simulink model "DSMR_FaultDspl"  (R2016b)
settings: Solver=FixedStepDiscrete  StartTime=0.0  StopTime=10.0  FixedStep=0.02  RelTol=1e-3  EnableMultiTasking=on
undefined symbols (not defined in the file): bin2dec
libraries: simulink x312
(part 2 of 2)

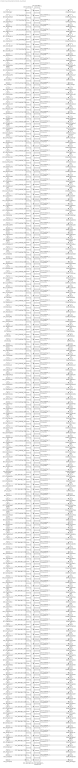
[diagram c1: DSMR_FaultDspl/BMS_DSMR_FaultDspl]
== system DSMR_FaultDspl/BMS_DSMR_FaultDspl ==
  DFC_CurrRngErr : Inport
  DFC_BattVoltRngErr : Inport  Port=2
  DFC_BattHVMsgTmt : Inport  Port=3
  DFC_BusHVMsgTmt : Inport  Port=4
  DFC_638LinCommErr : Inport  Port=5
  DFC_CellTempTmt : Inport  Port=6
  DFC_CellVoltTmt : Inport  Port=7
  DFC_InCanBusOff : Inport  Port=8
  DFC_VeCanBusOff : Inport  Port=9
  DFC_Msg2A3Tmt : Inport  Port=10
  DFC_RcMsg2A3Mis : Inport  Port=11
  DFC_ChkSumMsg2A3Err : Inport  Port=12
  DFC_RcMsg2A5Mis : Inport  Port=13
  DFC_RcMsg2A7Mis : Inport  Port=14
  DFC_CrashNpl : Inport  Port=15
  DFC_FuseNpl : Inport  Port=16
  DFC_Kl30cVoltLoErr : Inport  Port=17
  DFC_PosStuckMax : Inport  Port=18
  DFC_MPosStuckMin : Inport  Port=19
  DFC_MNegStuckMax : Inport  Port=20
  DFC_MNegStuckMin : Inport  Port=21
  DFC_PrStuckMin : Inport  Port=22
  DFC_DChrgPosStuckMax : Inport  Port=23
  DFC_DChrgPosStuckMin : Inport  Port=24
  DFC_DChrgNegStuckMax : Inport  Port=25
  DFC_DChrgNegStuckMin : Inport  Port=26
  DFC_HvPwrUpFail : Inport  Port=27
  DFC_DChrgPwrUpFail : Inport  Port=28
  DFC_BattTAlrmMax : Inport  Port=29
  DFC_BattTFaultMax : Inport  Port=30
  DFC_BattTAlrmMin : Inport  Port=31
  DFC_BattTFaultMin : Inport  Port=32
  DFC_BattTempVldMin : Inport  Port=33
  DFC_BattTCnstMax : Inport  Port=34
  DFC_BattTGradtMax : Inport  Port=35
  DFC_CellVoltAlrmMax : Inport  Port=36
  DFC_CellVoltFaultMax : Inport  Port=37
  DFC_CellVoltFusfMax : Inport  Port=38
  DFC_CellVoltAlrmMin : Inport  Port=39
  DFC_CellVoltFusfMin : Inport  Port=40
  DFC_CellVoltFaultMin : Inport  Port=41
  DFC_CellVoltVldMin : Inport  Port=42
  DFC_CellVoltNpl : Inport  Port=43
  DFC_Msg2E6Tmt : Inport  Port=44
  DFC_RcMsg2E6Mis : Inport  Port=45
  DFC_ChkSumMsg2E6Err : Inport  Port=46
  DFC_RcMsg2E1Mis : Inport  Port=47
  DFC_ChkSumMsg2E1Err : Inport  Port=48
  DFC_DcCanBusOff : Inport  Port=49
  DFC_DChrgTCnntMax : Inport  Port=50
  DFC_ChrgOCNpl : Inport  Port=51
  DFC_DisChOCNpl : Inport  Port=52
  DFC_BattVoltHiMax : Inport  Port=53
  DFC_BattVoltLoMin : Inport  Port=54
  DFC_ThmRnwy : Inport  Port=55
  DFC_AChrgPortOvrTemp : Inport  Port=56
  DFC_CurrOffsPlaus : Inport  Port=57
  DFC_CurrStukPlaus : Inport  Port=58
  DFC_CurrChrgPlaus : Inport  Port=59
  DFC_BattUNpl : Inport  Port=60
  DFC_BattVoltVld : Inport  Port=61
  DFC_PackUNpl : Inport  Port=62
  DFC_PackVoltVld : Inport  Port=63
  DFC_DChrgUNpl : Inport  Port=64
  DFC_DChrgVoltVld : Inport  Port=65
  DFC_BoardTempTmt : Inport  Port=66
  DFC_HvilMax : Inport  Port=67
  DFC_HvilMin : Inport  Port=68
  DFC_HvilSig : Inport  Port=69
  DFC_ChkSumMsg050Err : Inport  Port=70
  DFC_RcMsg050Mis : Inport  Port=71
  DFC_CrashHwNpl : Inport  Port=72
  DFC_IsoChkLv1 : Inport  Port=73
  DFC_IsoChkLv2 : Inport  Port=74
  DFC_InsResValdFault : Inport  Port=75
  DFC_Kl30OutRngErr : Inport  Port=76
  DFC_Kl30VoltLoErr : Inport  Port=77
  DFC_Kl30VoltHiErr : Inport  Port=78
  DFC_EepReadErr : Inport  Port=79
  DFC_BalStuckMax : Inport  Port=80
  DFC_BalStuckMin : Inport  Port=81
  DFC_CSCPwrSpyHiErr : Inport  Port=82
  DFC_CSCPwrSpyLoErr : Inport  Port=83
  DFC_CmcBordOTMax : Inport  Port=84
  DFC_BattTWarnMax : Inport  Port=85
  DFC_BattTWarnMin : Inport  Port=86
  DFC_BattTempVldMax : Inport  Port=87
  DFC_BattTHopMax : Inport  Port=88
  DFC_CellVoltRngHiErr : Inport  Port=89
  DFC_CellVoltRngLoErr : Inport  Port=90
  DFC_CellVoltWarnMax : Inport  Port=91
  DFC_CellVoltWarnMin : Inport  Port=92
  DFC_CellVoltVldMax : Inport  Port=93
  DFC_AChrgCurrMish : Inport  Port=94
  DFC_DChrgCurrMish : Inport  Port=95
  DFC_DChrgLowTempCurrMish : Inport  Port=96
  DFC_AChrgVoltMish : Inport  Port=97
  DFC_DChrgVoltMish : Inport  Port=98
  DFC_DChrgBattTMin : Inport  Port=99
  DFC_CC2Chk : Inport  Port=100
  DFC_APlusChk : Inport  Port=101
  DFC_DChrgMsgTmt : Inport  Port=102
  DFC_DChrgTNegElecMax : Inport  Port=103
  DFC_DChrgTNegElecMin : Inport  Port=104
  DFC_DChrgTNegElecSig : Inport  Port=105
  DFC_DChrgTPosElecMax : Inport  Port=106
  DFC_DChrgTPosElecMin : Inport  Port=107
  DFC_DChrgTPosElecSig : Inport  Port=108
  DFC_CcuSelfChkErr : Inport  Port=109
  DFC_ChrgOCMin : Inport  Port=110
  DFC_ChrgOCMax : Inport  Port=111
  DFC_DisChOCMin : Inport  Port=112
  DFC_DisChOCMax : Inport  Port=113
  DFC_SocRngLoMax : Inport  Port=114
  DFC_SocRngLoMin : Inport  Port=115
  DFC_SocRngHiMax : Inport  Port=116
  DFC_SocRngHiMin : Inport  Port=117
  DFC_InClntOverTmp : Inport  Port=118
  DFC_OutClntOverTmp : Inport  Port=119
  DFC_ClntDsTElecMax : Inport  Port=120
  DFC_ClntDsTElecMin : Inport  Port=121
  DFC_ClntDsTElecSig : Inport  Port=122
  DFC_ClntUsTElecMax : Inport  Port=123
  DFC_ClntUsTElecMin : Inport  Port=124
  DFC_ClntUsTElecSig : Inport  Port=125
  DFC_CoolPerfPlaus : Inport  Port=126
  DFC_HtgPerfPlaus : Inport  Port=127
  DFC_DChrgFobd : Inport  Port=128
  DFC_DChrgHvOnFail : Inport  Port=129
  DFC_AChgHVOnTmt : Inport  Port=130
  DFC_AChgHVOffTmt : Inport  Port=131
  DFC_AChgS2ClsdTmt : Inport  Port=132
  DFC_DChrgStakeErr : Inport  Port=133
  DFC_DChrgStkVoltErr : Inport  Port=134
  DFC_DChrgStkCurrErr : Inport  Port=135
  DFC_AChgPileRdyTmt : Inport  Port=136
  DFC_DChrgCHMTmt : Inport  Port=137
  DFC_DChrgCRMTmt : Inport  Port=138
  DFC_DChrgCMLTmt : Inport  Port=139
  DFC_DChrgCROTmt : Inport  Port=140
  DFC_DChrgCCSTmt : Inport  Port=141
  DFC_DChrgCSTTmt : Inport  Port=142
  DFC_DChrgCSDTmt : Inport  Port=143
  DFC_DChrgParaChk : Inport  Port=144
  DFC_DChrgCableChk : Inport  Port=145
  DFC_DChrgSLACTOut : Inport  Port=146
  DFC_DChrgCnntErr : Inport  Port=147
  DFC_DChrgLckErr : Inport  Port=148
  DFC_AChrgCnntErr : Inport  Port=149
  DFC_AChgLckTmt : Inport  Port=150
  DFC_AChgRdyPndiTmt : Inport  Port=151
  DFC_AChgRdyTmt : Inport  Port=152
  DFC_AChgingErr : Inport  Port=153
  DFC_AChgUnlckTmt : Inport  Port=154
  DFC_AChgFobd : Inport  Port=155
  DFC_SocValJmp : Inport  Port=156
  DFC_BattUNpl_{1..156} (156 alike) : simulink/Logic and Bit Operations/Bitwise Operator  logicop=AND  UseBitMask=on  BitMask=bin2dec('00011000')  BitMaskRealWorld=Stored Integer
  DFC_BattUNpl_1_compare{,1..155} (156 alike) : simulink/Logic and Bit Operations/Compare To Constant  relop===  const=24  OutDataTypeStr=boolean
  DSMR_CurrRngErr : Outport
  DSMR_BattVoltRngErr : Outport  Port=2
  DSMR_BattHVMsgTmt : Outport  Port=3
  DSMR_BusHVMsgTmt : Outport  Port=4
  DSMR_638LinCommErr : Outport  Port=5
  DSMR_CellTempTmt : Outport  Port=6
  DSMR_CellVoltTmt : Outport  Port=7
  DSMR_InCanBusOff : Outport  Port=8
  DSMR_VeCanBusOff : Outport  Port=9
  DSMR_Msg2A3Tmt : Outport  Port=10
  DSMR_RcMsg2A3Mis : Outport  Port=11
  DSMR_ChkSumMsg2A3Err : Outport  Port=12
  DSMR_RcMsg2A5Mis : Outport  Port=13
  DSMR_RcMsg2A7Mis : Outport  Port=14
  DSMR_CrashNpl : Outport  Port=15
  DSMR_FuseNpl : Outport  Port=16
  DSMR_Kl30cVoltLoErr : Outport  Port=17
  DSMR_PosStuckMax : Outport  Port=18
  DSMR_MPosStuckMin : Outport  Port=19
  DSMR_MNegStuckMax : Outport  Port=20
  DSMR_MNegStuckMin : Outport  Port=21
  DSMR_PrStuckMin : Outport  Port=22
  DSMR_DChrgPosStuckMax : Outport  Port=23
  DSMR_DChrgPosStuckMin : Outport  Port=24
  DSMR_DChrgNegStuckMax : Outport  Port=25
  DSMR_DChrgNegStuckMin : Outport  Port=26
  DSMR_HvPwrUpFail : Outport  Port=27
  DSMR_DChrgPwrUpFail : Outport  Port=28
  DSMR_BattTAlrmMax : Outport  Port=29
  DSMR_BattTFaultMax : Outport  Port=30
  DSMR_BattTAlrmMin : Outport  Port=31
  DSMR_BattTFaultMin : Outport  Port=32
  DSMR_BattTempVldMin : Outport  Port=33
  DSMR_BattTCnstMax : Outport  Port=34
  DSMR_BattTGradtMax : Outport  Port=35
  DSMR_CellVoltAlrmMax : Outport  Port=36
  DSMR_CellVoltFaultMax : Outport  Port=37
  DSMR_CellVoltFusfMax : Outport  Port=38
  DSMR_CellVoltAlrmMin : Outport  Port=39
  DSMR_CellVoltFusfMin : Outport  Port=40
  DSMR_CellVoltFaultMin : Outport  Port=41
  DSMR_CellVoltVldMin : Outport  Port=42
  DSMR_CellVoltNpl : Outport  Port=43
  DSMR_Msg2E6Tmt : Outport  Port=44
  DSMR_RcMsg2E6Mis : Outport  Port=45
  DSMR_ChkSumMsg2E6Err : Outport  Port=46
  DSMR_RcMsg2E1Mis : Outport  Port=47
  DSMR_ChkSumMsg2E1Err : Outport  Port=48
  DSMR_DcCanBusOff : Outport  Port=49
  DSMR_DChrgTCnntMax : Outport  Port=50
  DSMR_ChrgOCNpl : Outport  Port=51
  DSMR_DisChOCNpl : Outport  Port=52
  DSMR_BattVoltHiMax : Outport  Port=53
  DSMR_BattVoltLoMin : Outport  Port=54
  DSMR_ThmRnwy : Outport  Port=55
  DSMR_AChrgPortOvrTemp : Outport  Port=56
  DSMR_CurrOffsPlaus : Outport  Port=57
  DSMR_CurrStukPlaus : Outport  Port=58
  DSMR_CurrChrgPlaus : Outport  Port=59
  DSMR_BattUNpl : Outport  Port=60
  DSMR_BattVoltVld : Outport  Port=61
  DSMR_PackUNpl : Outport  Port=62
  DSMR_PackVoltVld : Outport  Port=63
  DSMR_DChrgUNpl : Outport  Port=64
  DSMR_DChrgVoltVld : Outport  Port=65
  DSMR_BoardTempTmt : Outport  Port=66
  DSMR_HvilMax : Outport  Port=67
  DSMR_HvilMin : Outport  Port=68
  DSMR_HvilSig : Outport  Port=69
  DSMR_ChkSumMsg050Err : Outport  Port=70
  DSMR_RcMsg050Mis : Outport  Port=71
  DSMR_CrashHwNpl : Outport  Port=72
  DSMR_IsoChkLv1 : Outport  Port=73
  DSMR_IsoChkLv2 : Outport  Port=74
  DSMR_InsResValdFault : Outport  Port=75
  DSMR_Kl30OutRngErr : Outport  Port=76
  DSMR_Kl30VoltLoErr : Outport  Port=77
  DSMR_Kl30VoltHiErr : Outport  Port=78
  DSMR_EepReadErr : Outport  Port=79
  DSMR_BalStuckMax : Outport  Port=80
  DSMR_BalStuckMin : Outport  Port=81
  DSMR_CSCPwrSpyHiErr : Outport  Port=82
  DSMR_CSCPwrSpyLoErr : Outport  Port=83
  DSMR_CmcBordOTMax : Outport  Port=84
  DSMR_BattTWarnMax : Outport  Port=85
  DSMR_BattTWarnMin : Outport  Port=86
  DSMR_BattTempVldMax : Outport  Port=87
  DSMR_BattTHopMax : Outport  Port=88
  DSMR_CellVoltRngHiErr : Outport  Port=89
  DSMR_CellVoltRngLoErr : Outport  Port=90
  DSMR_CellVoltWarnMax : Outport  Port=91
  DSMR_CellVoltWarnMin : Outport  Port=92
  DSMR_CellVoltVldMax : Outport  Port=93
  DSMR_AChrgCurrMish : Outport  Port=94
  DSMR_DChrgCurrMish : Outport  Port=95
  DSMR_DChrgLowTempCurrMish : Outport  Port=96
  DSMR_AChrgVoltMish : Outport  Port=97
  DSMR_DChrgVoltMish : Outport  Port=98
  DSMR_DChrgBattTMin : Outport  Port=99
  DSMR_CC2Chk : Outport  Port=100
  DSMR_APlusChk : Outport  Port=101
  DSMR_DChrgMsgTmt : Outport  Port=102
  DSMR_DChrgTNegElecMax : Outport  Port=103
  DSMR_DChrgTNegElecMin : Outport  Port=104
  DSMR_DChrgTNegElecSig : Outport  Port=105
  DSMR_DChrgTPosElecMax : Outport  Port=106
  DSMR_DChrgTPosElecMin : Outport  Port=107
  DSMR_DChrgTPosElecSig : Outport  Port=108
  DSMR_CcuSelfChkErr : Outport  Port=109
  DSMR_ChrgOCMin : Outport  Port=110
  DSMR_ChrgOCMax : Outport  Port=111
  DSMR_DisChOCMin : Outport  Port=112
  DSMR_DisChOCMax : Outport  Port=113
  DSMR_SocRngLoMax : Outport  Port=114
  DSMR_SocRngLoMin : Outport  Port=115
  DSMR_SocRngHiMax : Outport  Port=116
  DSMR_SocRngHiMin : Outport  Port=117
  DSMR_InClntOverTmp : Outport  Port=118
  DSMR_OutClntOverTmp : Outport  Port=119
  DSMR_ClntDsTElecMax : Outport  Port=120
  DSMR_ClntDsTElecMin : Outport  Port=121
  DSMR_ClntDsTElecSig : Outport  Port=122
  DSMR_ClntUsTElecMax : Outport  Port=123
  DSMR_ClntUsTElecMin : Outport  Port=124
  DSMR_ClntUsTElecSig : Outport  Port=125
  DSMR_CoolPerfPlaus : Outport  Port=126
  DSMR_HtgPerfPlaus : Outport  Port=127
  DSMR_DChrgFobd : Outport  Port=128
  DSMR_DChrgHvOnFail : Outport  Port=129
  DSMR_AChgHVOnTmt : Outport  Port=130
  DSMR_AChgHVOffTmt : Outport  Port=131
  DSMR_AChgS2ClsdTmt : Outport  Port=132
  DSMR_DChrgStakeErr : Outport  Port=133
  DSMR_DChrgStkVoltErr : Outport  Port=134
  DSMR_DChrgStkCurrErr : Outport  Port=135
  DSMR_AChgPileRdyTmt : Outport  Port=136
  DSMR_DChrgCHMTmt : Outport  Port=137
  DSMR_DChrgCRMTmt : Outport  Port=138
  DSMR_DChrgCMLTmt : Outport  Port=139
  DSMR_DChrgCROTmt : Outport  Port=140
  DSMR_DChrgCCSTmt : Outport  Port=141
  DSMR_DChrgCSTTmt : Outport  Port=142
  DSMR_DChrgCSDTmt : Outport  Port=143
  DSMR_DChrgParaChk : Outport  Port=144
  DSMR_DChrgCableChk : Outport  Port=145
  DSMR_DChrgSLACTOut : Outport  Port=146
  DSMR_DChrgCnntErr : Outport  Port=147
  DSMR_DChrgLckErr : Outport  Port=148
  DSMR_AChrgCnntErr : Outport  Port=149
  DSMR_AChgLckTmt : Outport  Port=150
  DSMR_AChgRdyPndiTmt : Outport  Port=151
  DSMR_AChgRdyTmt : Outport  Port=152
  DSMR_AChgingErr : Outport  Port=153
  DSMR_AChgUnlckTmt : Outport  Port=154
  DSMR_AChgFobd : Outport  Port=155
  DSMR_SocValJmp : Outport  Port=156
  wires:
  DFC_CurrRngErr/1 -> DFC_BattUNpl_1/1
  DFC_BattUNpl_2/1 -> DFC_BattUNpl_1_compare1/1
  DFC_BattVoltRngErr/1 -> DFC_BattUNpl_2/1
  DFC_BattUNpl_1_compare1/1 -> DSMR_BattVoltRngErr/1
  DFC_BattUNpl_3/1 -> DFC_BattUNpl_1_compare2/1
  DFC_BattHVMsgTmt/1 -> DFC_BattUNpl_3/1
  DFC_BattUNpl_1_compare2/1 -> DSMR_BattHVMsgTmt/1
  DFC_BattUNpl_4/1 -> DFC_BattUNpl_1_compare3/1
  DFC_BusHVMsgTmt/1 -> DFC_BattUNpl_4/1
  DFC_BattUNpl_1_compare3/1 -> DSMR_BusHVMsgTmt/1
  DFC_BattUNpl_5/1 -> DFC_BattUNpl_1_compare4/1
  DFC_638LinCommErr/1 -> DFC_BattUNpl_5/1
  DFC_BattUNpl_1_compare4/1 -> DSMR_638LinCommErr/1
  DFC_BattUNpl_6/1 -> DFC_BattUNpl_1_compare5/1
  DFC_CellTempTmt/1 -> DFC_BattUNpl_6/1
  DFC_BattUNpl_1_compare5/1 -> DSMR_CellTempTmt/1
  DFC_BattUNpl_7/1 -> DFC_BattUNpl_1_compare6/1
  DFC_CellVoltTmt/1 -> DFC_BattUNpl_7/1
  DFC_BattUNpl_1_compare6/1 -> DSMR_CellVoltTmt/1
  DFC_BattUNpl_8/1 -> DFC_BattUNpl_1_compare7/1
  DFC_InCanBusOff/1 -> DFC_BattUNpl_8/1
  DFC_BattUNpl_1_compare7/1 -> DSMR_InCanBusOff/1
  DFC_BattUNpl_9/1 -> DFC_BattUNpl_1_compare8/1
  DFC_VeCanBusOff/1 -> DFC_BattUNpl_9/1
  DFC_BattUNpl_1_compare8/1 -> DSMR_VeCanBusOff/1
  DFC_BattUNpl_10/1 -> DFC_BattUNpl_1_compare9/1
  DFC_Msg2A3Tmt/1 -> DFC_BattUNpl_10/1
  DFC_BattUNpl_1_compare9/1 -> DSMR_Msg2A3Tmt/1
  DFC_BattUNpl_11/1 -> DFC_BattUNpl_1_compare10/1
  DFC_RcMsg2A3Mis/1 -> DFC_BattUNpl_11/1
  DFC_BattUNpl_1_compare10/1 -> DSMR_RcMsg2A3Mis/1
  DFC_BattUNpl_12/1 -> DFC_BattUNpl_1_compare11/1
  DFC_ChkSumMsg2A3Err/1 -> DFC_BattUNpl_12/1
  DFC_BattUNpl_1_compare11/1 -> DSMR_ChkSumMsg2A3Err/1
  DFC_BattUNpl_13/1 -> DFC_BattUNpl_1_compare12/1
  DFC_RcMsg2A5Mis/1 -> DFC_BattUNpl_13/1
  DFC_BattUNpl_1_compare12/1 -> DSMR_RcMsg2A5Mis/1
  DFC_BattUNpl_14/1 -> DFC_BattUNpl_1_compare13/1
  DFC_RcMsg2A7Mis/1 -> DFC_BattUNpl_14/1
  DFC_BattUNpl_1_compare13/1 -> DSMR_RcMsg2A7Mis/1
  DFC_BattUNpl_15/1 -> DFC_BattUNpl_1_compare14/1
  DFC_CrashNpl/1 -> DFC_BattUNpl_15/1
  DFC_BattUNpl_1_compare14/1 -> DSMR_CrashNpl/1
  DFC_BattUNpl_16/1 -> DFC_BattUNpl_1_compare15/1
  DFC_FuseNpl/1 -> DFC_BattUNpl_16/1
  DFC_BattUNpl_1_compare15/1 -> DSMR_FuseNpl/1
  DFC_BattUNpl_17/1 -> DFC_BattUNpl_1_compare16/1
  DFC_Kl30cVoltLoErr/1 -> DFC_BattUNpl_17/1
  DFC_BattUNpl_1_compare16/1 -> DSMR_Kl30cVoltLoErr/1
  DFC_BattUNpl_25/1 -> DFC_BattUNpl_1_compare17/1
  DFC_PosStuckMax/1 -> DFC_BattUNpl_25/1
  DFC_BattUNpl_1_compare17/1 -> DSMR_PosStuckMax/1
  DFC_BattUNpl_26/1 -> DFC_BattUNpl_1_compare24/1
  DFC_MPosStuckMin/1 -> DFC_BattUNpl_26/1
  DFC_BattUNpl_1_compare24/1 -> DSMR_MPosStuckMin/1
  DFC_BattUNpl_27/1 -> DFC_BattUNpl_1_compare25/1
  DFC_MNegStuckMax/1 -> DFC_BattUNpl_27/1
  DFC_BattUNpl_1_compare25/1 -> DSMR_MNegStuckMax/1
  DFC_BattUNpl_28/1 -> DFC_BattUNpl_1_compare26/1
  DFC_MNegStuckMin/1 -> DFC_BattUNpl_28/1
  DFC_BattUNpl_1_compare26/1 -> DSMR_MNegStuckMin/1
  DFC_BattUNpl_29/1 -> DFC_BattUNpl_1_compare27/1
  DFC_PrStuckMin/1 -> DFC_BattUNpl_29/1
  DFC_BattUNpl_1_compare27/1 -> DSMR_PrStuckMin/1
  DFC_BattUNpl_30/1 -> DFC_BattUNpl_1_compare28/1
  DFC_DChrgPosStuckMax/1 -> DFC_BattUNpl_30/1
  DFC_BattUNpl_1_compare28/1 -> DSMR_DChrgPosStuckMax/1
  DFC_BattUNpl_31/1 -> DFC_BattUNpl_1_compare29/1
  DFC_DChrgPosStuckMin/1 -> DFC_BattUNpl_31/1
  DFC_BattUNpl_1_compare29/1 -> DSMR_DChrgPosStuckMin/1
  DFC_BattUNpl_32/1 -> DFC_BattUNpl_1_compare30/1
  DFC_DChrgNegStuckMax/1 -> DFC_BattUNpl_32/1
  DFC_BattUNpl_1_compare30/1 -> DSMR_DChrgNegStuckMax/1
  DFC_BattUNpl_18/1 -> DFC_BattUNpl_1_compare31/1
  DFC_DChrgNegStuckMin/1 -> DFC_BattUNpl_18/1
  DFC_BattUNpl_1_compare31/1 -> DSMR_DChrgNegStuckMin/1
  DFC_BattUNpl_19/1 -> DFC_BattUNpl_1_compare18/1
  DFC_HvPwrUpFail/1 -> DFC_BattUNpl_19/1
  DFC_BattUNpl_1_compare18/1 -> DSMR_HvPwrUpFail/1
  DFC_BattUNpl_20/1 -> DFC_BattUNpl_1_compare19/1
  DFC_DChrgPwrUpFail/1 -> DFC_BattUNpl_20/1
  DFC_BattUNpl_1_compare19/1 -> DSMR_DChrgPwrUpFail/1
  DFC_BattUNpl_21/1 -> DFC_BattUNpl_1_compare20/1
  DFC_BattTAlrmMax/1 -> DFC_BattUNpl_21/1
  DFC_BattUNpl_1_compare20/1 -> DSMR_BattTAlrmMax/1
  DFC_BattUNpl_22/1 -> DFC_BattUNpl_1_compare21/1
  DFC_BattTFaultMax/1 -> DFC_BattUNpl_22/1
  DFC_BattUNpl_1_compare21/1 -> DSMR_BattTFaultMax/1
  DFC_BattUNpl_23/1 -> DFC_BattUNpl_1_compare22/1
  DFC_BattTAlrmMin/1 -> DFC_BattUNpl_23/1
  DFC_BattUNpl_1_compare22/1 -> DSMR_BattTAlrmMin/1
  DFC_BattUNpl_24/1 -> DFC_BattUNpl_1_compare23/1
  DFC_BattTFaultMin/1 -> DFC_BattUNpl_24/1
  DFC_BattUNpl_1_compare23/1 -> DSMR_BattTFaultMin/1
  DFC_BattUNpl_33/1 -> DFC_BattUNpl_1_compare32/1
  DFC_BattTempVldMin/1 -> DFC_BattUNpl_33/1
  DFC_BattUNpl_1_compare32/1 -> DSMR_BattTempVldMin/1
  DFC_BattUNpl_41/1 -> DFC_BattUNpl_1_compare33/1
  DFC_BattTCnstMax/1 -> DFC_BattUNpl_41/1
  DFC_BattUNpl_1_compare33/1 -> DSMR_BattTCnstMax/1
  DFC_BattUNpl_42/1 -> DFC_BattUNpl_1_compare40/1
  DFC_BattTGradtMax/1 -> DFC_BattUNpl_42/1
  DFC_BattUNpl_1_compare40/1 -> DSMR_BattTGradtMax/1
  DFC_BattUNpl_43/1 -> DFC_BattUNpl_1_compare41/1
  DFC_CellVoltAlrmMax/1 -> DFC_BattUNpl_43/1
  DFC_BattUNpl_1_compare41/1 -> DSMR_CellVoltAlrmMax/1
  DFC_BattUNpl_44/1 -> DFC_BattUNpl_1_compare42/1
  DFC_CellVoltFaultMax/1 -> DFC_BattUNpl_44/1
  DFC_BattUNpl_1_compare42/1 -> DSMR_CellVoltFaultMax/1
  DFC_BattUNpl_45/1 -> DFC_BattUNpl_1_compare43/1
  DFC_CellVoltFusfMax/1 -> DFC_BattUNpl_45/1
  DFC_BattUNpl_1_compare43/1 -> DSMR_CellVoltFusfMax/1
  DFC_BattUNpl_46/1 -> DFC_BattUNpl_1_compare44/1
  DFC_CellVoltAlrmMin/1 -> DFC_BattUNpl_46/1
  DFC_BattUNpl_1_compare44/1 -> DSMR_CellVoltAlrmMin/1
  DFC_BattUNpl_47/1 -> DFC_BattUNpl_1_compare45/1
  DFC_CellVoltFusfMin/1 -> DFC_BattUNpl_47/1
  DFC_BattUNpl_1_compare45/1 -> DSMR_CellVoltFusfMin/1
  DFC_BattUNpl_48/1 -> DFC_BattUNpl_1_compare46/1
  DFC_CellVoltFaultMin/1 -> DFC_BattUNpl_48/1
  DFC_BattUNpl_1_compare46/1 -> DSMR_CellVoltFaultMin/1
  DFC_BattUNpl_34/1 -> DFC_BattUNpl_1_compare47/1
  DFC_CellVoltVldMin/1 -> DFC_BattUNpl_34/1
  DFC_BattUNpl_1_compare47/1 -> DSMR_CellVoltVldMin/1
  DFC_BattUNpl_35/1 -> DFC_BattUNpl_1_compare34/1
  DFC_CellVoltNpl/1 -> DFC_BattUNpl_35/1
  DFC_BattUNpl_1_compare34/1 -> DSMR_CellVoltNpl/1
  DFC_BattUNpl_36/1 -> DFC_BattUNpl_1_compare35/1
  DFC_Msg2E6Tmt/1 -> DFC_BattUNpl_36/1
  DFC_BattUNpl_1_compare35/1 -> DSMR_Msg2E6Tmt/1
  DFC_BattUNpl_37/1 -> DFC_BattUNpl_1_compare36/1
  DFC_RcMsg2E6Mis/1 -> DFC_BattUNpl_37/1
  DFC_BattUNpl_1_compare36/1 -> DSMR_RcMsg2E6Mis/1
  DFC_BattUNpl_38/1 -> DFC_BattUNpl_1_compare37/1
  DFC_ChkSumMsg2E6Err/1 -> DFC_BattUNpl_38/1
  DFC_BattUNpl_1_compare37/1 -> DSMR_ChkSumMsg2E6Err/1
  DFC_BattUNpl_39/1 -> DFC_BattUNpl_1_compare38/1
  DFC_RcMsg2E1Mis/1 -> DFC_BattUNpl_39/1
  DFC_BattUNpl_1_compare38/1 -> DSMR_RcMsg2E1Mis/1
  DFC_BattUNpl_40/1 -> DFC_BattUNpl_1_compare39/1
  DFC_ChkSumMsg2E1Err/1 -> DFC_BattUNpl_40/1
  DFC_BattUNpl_1_compare39/1 -> DSMR_ChkSumMsg2E1Err/1
  DFC_BattUNpl_49/1 -> DFC_BattUNpl_1_compare48/1
  DFC_DcCanBusOff/1 -> DFC_BattUNpl_49/1
  DFC_BattUNpl_1_compare48/1 -> DSMR_DcCanBusOff/1
  DFC_BattUNpl_57/1 -> DFC_BattUNpl_1_compare49/1
  DFC_DChrgTCnntMax/1 -> DFC_BattUNpl_57/1
  DFC_BattUNpl_1_compare49/1 -> DSMR_DChrgTCnntMax/1
  DFC_BattUNpl_58/1 -> DFC_BattUNpl_1_compare56/1
  DFC_ChrgOCNpl/1 -> DFC_BattUNpl_58/1
  DFC_BattUNpl_1_compare56/1 -> DSMR_ChrgOCNpl/1
  DFC_BattUNpl_59/1 -> DFC_BattUNpl_1_compare57/1
  DFC_DisChOCNpl/1 -> DFC_BattUNpl_59/1
  DFC_BattUNpl_1_compare57/1 -> DSMR_DisChOCNpl/1
  DFC_BattUNpl_60/1 -> DFC_BattUNpl_1_compare58/1
  DFC_BattVoltHiMax/1 -> DFC_BattUNpl_60/1
  DFC_BattUNpl_1_compare58/1 -> DSMR_BattVoltHiMax/1
  DFC_BattUNpl_61/1 -> DFC_BattUNpl_1_compare59/1
  DFC_BattVoltLoMin/1 -> DFC_BattUNpl_61/1
  DFC_BattUNpl_1_compare59/1 -> DSMR_BattVoltLoMin/1
  DFC_BattUNpl_62/1 -> DFC_BattUNpl_1_compare60/1
  DFC_ThmRnwy/1 -> DFC_BattUNpl_62/1
  DFC_BattUNpl_1_compare60/1 -> DSMR_ThmRnwy/1
  DFC_BattUNpl_63/1 -> DFC_BattUNpl_1_compare61/1
  DFC_AChrgPortOvrTemp/1 -> DFC_BattUNpl_63/1
  DFC_BattUNpl_1_compare61/1 -> DSMR_AChrgPortOvrTemp/1
  DFC_BattUNpl_64/1 -> DFC_BattUNpl_1_compare62/1
  DFC_CurrOffsPlaus/1 -> DFC_BattUNpl_64/1
  DFC_BattUNpl_1_compare62/1 -> DSMR_CurrOffsPlaus/1
  DFC_BattUNpl_50/1 -> DFC_BattUNpl_1_compare63/1
  DFC_CurrStukPlaus/1 -> DFC_BattUNpl_50/1
  DFC_BattUNpl_1_compare63/1 -> DSMR_CurrStukPlaus/1
  DFC_BattUNpl_51/1 -> DFC_BattUNpl_1_compare50/1
  DFC_CurrChrgPlaus/1 -> DFC_BattUNpl_51/1
  DFC_BattUNpl_1_compare50/1 -> DSMR_CurrChrgPlaus/1
  DFC_BattUNpl_52/1 -> DFC_BattUNpl_1_compare51/1
  DFC_BattUNpl/1 -> DFC_BattUNpl_52/1
  DFC_BattUNpl_1_compare51/1 -> DSMR_BattUNpl/1
  DFC_BattUNpl_53/1 -> DFC_BattUNpl_1_compare52/1
  DFC_BattVoltVld/1 -> DFC_BattUNpl_53/1
  DFC_BattUNpl_1_compare52/1 -> DSMR_BattVoltVld/1
  DFC_BattUNpl_54/1 -> DFC_BattUNpl_1_compare53/1
  DFC_PackUNpl/1 -> DFC_BattUNpl_54/1
  DFC_BattUNpl_1_compare53/1 -> DSMR_PackUNpl/1
  DFC_BattUNpl_55/1 -> DFC_BattUNpl_1_compare54/1
  DFC_PackVoltVld/1 -> DFC_BattUNpl_55/1
  DFC_BattUNpl_1_compare54/1 -> DSMR_PackVoltVld/1
  DFC_BattUNpl_56/1 -> DFC_BattUNpl_1_compare55/1
  DFC_DChrgUNpl/1 -> DFC_BattUNpl_56/1
  DFC_BattUNpl_1_compare55/1 -> DSMR_DChrgUNpl/1
  DFC_BattUNpl_65/1 -> DFC_BattUNpl_1_compare64/1
  DFC_DChrgVoltVld/1 -> DFC_BattUNpl_65/1
  DFC_BattUNpl_1_compare64/1 -> DSMR_DChrgVoltVld/1
  DFC_BattUNpl_73/1 -> DFC_BattUNpl_1_compare65/1
  DFC_BoardTempTmt/1 -> DFC_BattUNpl_73/1
  DFC_BattUNpl_1_compare65/1 -> DSMR_BoardTempTmt/1
  DFC_BattUNpl_74/1 -> DFC_BattUNpl_1_compare72/1
  DFC_HvilMax/1 -> DFC_BattUNpl_74/1
  DFC_BattUNpl_1_compare72/1 -> DSMR_HvilMax/1
  DFC_BattUNpl_75/1 -> DFC_BattUNpl_1_compare73/1
  DFC_HvilMin/1 -> DFC_BattUNpl_75/1
  DFC_BattUNpl_1_compare73/1 -> DSMR_HvilMin/1
  DFC_BattUNpl_76/1 -> DFC_BattUNpl_1_compare74/1
  DFC_HvilSig/1 -> DFC_BattUNpl_76/1
  DFC_BattUNpl_1_compare74/1 -> DSMR_HvilSig/1
  DFC_BattUNpl_77/1 -> DFC_BattUNpl_1_compare75/1
  DFC_ChkSumMsg050Err/1 -> DFC_BattUNpl_77/1
  DFC_BattUNpl_1_compare75/1 -> DSMR_ChkSumMsg050Err/1
  DFC_BattUNpl_78/1 -> DFC_BattUNpl_1_compare76/1
  DFC_RcMsg050Mis/1 -> DFC_BattUNpl_78/1
  DFC_BattUNpl_1_compare76/1 -> DSMR_RcMsg050Mis/1
  DFC_BattUNpl_79/1 -> DFC_BattUNpl_1_compare77/1
  DFC_CrashHwNpl/1 -> DFC_BattUNpl_79/1
  DFC_BattUNpl_1_compare77/1 -> DSMR_CrashHwNpl/1
  DFC_BattUNpl_80/1 -> DFC_BattUNpl_1_compare78/1
  DFC_IsoChkLv1/1 -> DFC_BattUNpl_80/1
  DFC_BattUNpl_1_compare78/1 -> DSMR_IsoChkLv1/1
  DFC_BattUNpl_66/1 -> DFC_BattUNpl_1_compare79/1
  DFC_IsoChkLv2/1 -> DFC_BattUNpl_66/1
  DFC_BattUNpl_1_compare79/1 -> DSMR_IsoChkLv2/1
  DFC_BattUNpl_67/1 -> DFC_BattUNpl_1_compare66/1
  DFC_InsResValdFault/1 -> DFC_BattUNpl_67/1
  DFC_BattUNpl_1_compare66/1 -> DSMR_InsResValdFault/1
  DFC_BattUNpl_68/1 -> DFC_BattUNpl_1_compare67/1
  DFC_Kl30OutRngErr/1 -> DFC_BattUNpl_68/1
  DFC_BattUNpl_1_compare67/1 -> DSMR_Kl30OutRngErr/1
  DFC_BattUNpl_69/1 -> DFC_BattUNpl_1_compare68/1
  DFC_Kl30VoltLoErr/1 -> DFC_BattUNpl_69/1
  DFC_BattUNpl_1_compare68/1 -> DSMR_Kl30VoltLoErr/1
  DFC_BattUNpl_70/1 -> DFC_BattUNpl_1_compare69/1
  DFC_Kl30VoltHiErr/1 -> DFC_BattUNpl_70/1
  DFC_BattUNpl_1_compare69/1 -> DSMR_Kl30VoltHiErr/1
  DFC_BattUNpl_71/1 -> DFC_BattUNpl_1_compare70/1
  DFC_EepReadErr/1 -> DFC_BattUNpl_71/1
  DFC_BattUNpl_1_compare70/1 -> DSMR_EepReadErr/1
  DFC_BattUNpl_72/1 -> DFC_BattUNpl_1_compare71/1
  DFC_BalStuckMax/1 -> DFC_BattUNpl_72/1
  DFC_BattUNpl_1_compare71/1 -> DSMR_BalStuckMax/1
  DFC_BattUNpl_88/1 -> DFC_BattUNpl_1_compare80/1
  DFC_BalStuckMin/1 -> DFC_BattUNpl_88/1
  DFC_BattUNpl_1_compare80/1 -> DSMR_BalStuckMin/1
  DFC_BattUNpl_89/1 -> DFC_BattUNpl_1_compare87/1
  DFC_CSCPwrSpyHiErr/1 -> DFC_BattUNpl_89/1
  DFC_BattUNpl_1_compare87/1 -> DSMR_CSCPwrSpyHiErr/1
  DFC_BattUNpl_90/1 -> DFC_BattUNpl_1_compare88/1
  DFC_CSCPwrSpyLoErr/1 -> DFC_BattUNpl_90/1
  DFC_BattUNpl_1_compare88/1 -> DSMR_CSCPwrSpyLoErr/1
  DFC_BattUNpl_91/1 -> DFC_BattUNpl_1_compare89/1
  DFC_CmcBordOTMax/1 -> DFC_BattUNpl_91/1
  DFC_BattUNpl_1_compare89/1 -> DSMR_CmcBordOTMax/1
  DFC_BattUNpl_92/1 -> DFC_BattUNpl_1_compare90/1
  DFC_BattTWarnMax/1 -> DFC_BattUNpl_92/1
  DFC_BattUNpl_1_compare90/1 -> DSMR_BattTWarnMax/1
  DFC_BattUNpl_93/1 -> DFC_BattUNpl_1_compare91/1
  DFC_BattTWarnMin/1 -> DFC_BattUNpl_93/1
  DFC_BattUNpl_1_compare91/1 -> DSMR_BattTWarnMin/1
  DFC_BattUNpl_94/1 -> DFC_BattUNpl_1_compare92/1
  DFC_BattTempVldMax/1 -> DFC_BattUNpl_94/1
  DFC_BattUNpl_1_compare92/1 -> DSMR_BattTempVldMax/1
  DFC_BattUNpl_95/1 -> DFC_BattUNpl_1_compare93/1
  DFC_BattTHopMax/1 -> DFC_BattUNpl_95/1
  DFC_BattUNpl_1_compare93/1 -> DSMR_BattTHopMax/1
  DFC_BattUNpl_81/1 -> DFC_BattUNpl_1_compare94/1
  DFC_CellVoltRngHiErr/1 -> DFC_BattUNpl_81/1
  DFC_BattUNpl_1_compare94/1 -> DSMR_CellVoltRngHiErr/1
  DFC_BattUNpl_82/1 -> DFC_BattUNpl_1_compare81/1
  DFC_CellVoltRngLoErr/1 -> DFC_BattUNpl_82/1
  DFC_BattUNpl_1_compare81/1 -> DSMR_CellVoltRngLoErr/1
  DFC_BattUNpl_83/1 -> DFC_BattUNpl_1_compare82/1
  DFC_CellVoltWarnMax/1 -> DFC_BattUNpl_83/1
  DFC_BattUNpl_1_compare82/1 -> DSMR_CellVoltWarnMax/1
  DFC_BattUNpl_84/1 -> DFC_BattUNpl_1_compare83/1
  DFC_CellVoltWarnMin/1 -> DFC_BattUNpl_84/1
  DFC_BattUNpl_1_compare83/1 -> DSMR_CellVoltWarnMin/1
  DFC_BattUNpl_85/1 -> DFC_BattUNpl_1_compare84/1
  DFC_CellVoltVldMax/1 -> DFC_BattUNpl_85/1
  DFC_BattUNpl_1_compare84/1 -> DSMR_CellVoltVldMax/1
  DFC_BattUNpl_86/1 -> DFC_BattUNpl_1_compare85/1
  DFC_AChrgCurrMish/1 -> DFC_BattUNpl_86/1
  DFC_BattUNpl_1_compare85/1 -> DSMR_AChrgCurrMish/1
  DFC_BattUNpl_87/1 -> DFC_BattUNpl_1_compare86/1
  DFC_DChrgCurrMish/1 -> DFC_BattUNpl_87/1
  DFC_BattUNpl_1_compare86/1 -> DSMR_DChrgCurrMish/1
  DFC_BattUNpl_96/1 -> DFC_BattUNpl_1_compare95/1
  DFC_DChrgLowTempCurrMish/1 -> DFC_BattUNpl_96/1
  DFC_BattUNpl_1_compare95/1 -> DSMR_DChrgLowTempCurrMish/1
  DFC_BattUNpl_104/1 -> DFC_BattUNpl_1_compare96/1
  DFC_AChrgVoltMish/1 -> DFC_BattUNpl_104/1
  DFC_BattUNpl_1_compare96/1 -> DSMR_AChrgVoltMish/1
  DFC_BattUNpl_105/1 -> DFC_BattUNpl_1_compare103/1
  DFC_DChrgVoltMish/1 -> DFC_BattUNpl_105/1
  DFC_BattUNpl_1_compare103/1 -> DSMR_DChrgVoltMish/1
  DFC_BattUNpl_106/1 -> DFC_BattUNpl_1_compare104/1
  DFC_DChrgBattTMin/1 -> DFC_BattUNpl_106/1
  DFC_BattUNpl_1_compare104/1 -> DSMR_DChrgBattTMin/1
  DFC_BattUNpl_107/1 -> DFC_BattUNpl_1_compare105/1
  DFC_CC2Chk/1 -> DFC_BattUNpl_107/1
  DFC_BattUNpl_1_compare105/1 -> DSMR_CC2Chk/1
  DFC_BattUNpl_108/1 -> DFC_BattUNpl_1_compare106/1
  DFC_APlusChk/1 -> DFC_BattUNpl_108/1
  DFC_BattUNpl_1_compare106/1 -> DSMR_APlusChk/1
  DFC_BattUNpl_109/1 -> DFC_BattUNpl_1_compare107/1
  DFC_DChrgMsgTmt/1 -> DFC_BattUNpl_109/1
  DFC_BattUNpl_1_compare107/1 -> DSMR_DChrgMsgTmt/1
  DFC_BattUNpl_110/1 -> DFC_BattUNpl_1_compare108/1
  DFC_DChrgTNegElecMax/1 -> DFC_BattUNpl_110/1
  DFC_BattUNpl_1_compare108/1 -> DSMR_DChrgTNegElecMax/1
  DFC_BattUNpl_111/1 -> DFC_BattUNpl_1_compare109/1
  DFC_DChrgTNegElecMin/1 -> DFC_BattUNpl_111/1
  DFC_BattUNpl_1_compare109/1 -> DSMR_DChrgTNegElecMin/1
  DFC_BattUNpl_97/1 -> DFC_BattUNpl_1_compare110/1
  DFC_DChrgTNegElecSig/1 -> DFC_BattUNpl_97/1
  DFC_BattUNpl_1_compare110/1 -> DSMR_DChrgTNegElecSig/1
  DFC_BattUNpl_98/1 -> DFC_BattUNpl_1_compare97/1
  DFC_DChrgTPosElecMax/1 -> DFC_BattUNpl_98/1
  DFC_BattUNpl_1_compare97/1 -> DSMR_DChrgTPosElecMax/1
  DFC_BattUNpl_99/1 -> DFC_BattUNpl_1_compare98/1
  DFC_DChrgTPosElecMin/1 -> DFC_BattUNpl_99/1
  DFC_BattUNpl_1_compare98/1 -> DSMR_DChrgTPosElecMin/1
  DFC_BattUNpl_100/1 -> DFC_BattUNpl_1_compare99/1
  DFC_DChrgTPosElecSig/1 -> DFC_BattUNpl_100/1
  DFC_BattUNpl_1_compare99/1 -> DSMR_DChrgTPosElecSig/1
  DFC_BattUNpl_101/1 -> DFC_BattUNpl_1_compare100/1
  DFC_CcuSelfChkErr/1 -> DFC_BattUNpl_101/1
  DFC_BattUNpl_1_compare100/1 -> DSMR_CcuSelfChkErr/1
  DFC_BattUNpl_102/1 -> DFC_BattUNpl_1_compare101/1
  DFC_ChrgOCMin/1 -> DFC_BattUNpl_102/1
  DFC_BattUNpl_1_compare101/1 -> DSMR_ChrgOCMin/1
  DFC_BattUNpl_103/1 -> DFC_BattUNpl_1_compare102/1
  DFC_ChrgOCMax/1 -> DFC_BattUNpl_103/1
  DFC_BattUNpl_1_compare102/1 -> DSMR_ChrgOCMax/1
  DFC_BattUNpl_119/1 -> DFC_BattUNpl_1_compare111/1
  DFC_DisChOCMin/1 -> DFC_BattUNpl_119/1
  DFC_BattUNpl_1_compare111/1 -> DSMR_DisChOCMin/1
  DFC_BattUNpl_120/1 -> DFC_BattUNpl_1_compare118/1
  DFC_DisChOCMax/1 -> DFC_BattUNpl_120/1
  DFC_BattUNpl_1_compare118/1 -> DSMR_DisChOCMax/1
  DFC_BattUNpl_121/1 -> DFC_BattUNpl_1_compare119/1
  DFC_SocRngLoMax/1 -> DFC_BattUNpl_121/1
  DFC_BattUNpl_1_compare119/1 -> DSMR_SocRngLoMax/1
  DFC_BattUNpl_122/1 -> DFC_BattUNpl_1_compare120/1
  DFC_SocRngLoMin/1 -> DFC_BattUNpl_122/1
  DFC_BattUNpl_1_compare120/1 -> DSMR_SocRngLoMin/1
  DFC_BattUNpl_123/1 -> DFC_BattUNpl_1_compare121/1
  DFC_SocRngHiMax/1 -> DFC_BattUNpl_123/1
  DFC_BattUNpl_1_compare121/1 -> DSMR_SocRngHiMax/1
  DFC_BattUNpl_124/1 -> DFC_BattUNpl_1_compare122/1
  DFC_SocRngHiMin/1 -> DFC_BattUNpl_124/1
  DFC_BattUNpl_1_compare122/1 -> DSMR_SocRngHiMin/1
  DFC_BattUNpl_125/1 -> DFC_BattUNpl_1_compare123/1
  DFC_InClntOverTmp/1 -> DFC_BattUNpl_125/1
  DFC_BattUNpl_1_compare123/1 -> DSMR_InClntOverTmp/1
  DFC_BattUNpl_126/1 -> DFC_BattUNpl_1_compare124/1
  DFC_OutClntOverTmp/1 -> DFC_BattUNpl_126/1
  DFC_BattUNpl_1_compare124/1 -> DSMR_OutClntOverTmp/1
  DFC_BattUNpl_112/1 -> DFC_BattUNpl_1_compare125/1
  DFC_ClntDsTElecMax/1 -> DFC_BattUNpl_112/1
  DFC_BattUNpl_1_compare125/1 -> DSMR_ClntDsTElecMax/1
  DFC_BattUNpl_113/1 -> DFC_BattUNpl_1_compare112/1
  DFC_ClntDsTElecMin/1 -> DFC_BattUNpl_113/1
  DFC_BattUNpl_1_compare112/1 -> DSMR_ClntDsTElecMin/1
  DFC_BattUNpl_114/1 -> DFC_BattUNpl_1_compare113/1
  DFC_ClntDsTElecSig/1 -> DFC_BattUNpl_114/1
  DFC_BattUNpl_1_compare113/1 -> DSMR_ClntDsTElecSig/1
  DFC_BattUNpl_115/1 -> DFC_BattUNpl_1_compare114/1
  DFC_ClntUsTElecMax/1 -> DFC_BattUNpl_115/1
  DFC_BattUNpl_1_compare114/1 -> DSMR_ClntUsTElecMax/1
  DFC_BattUNpl_116/1 -> DFC_BattUNpl_1_compare115/1
  DFC_ClntUsTElecMin/1 -> DFC_BattUNpl_116/1
  DFC_BattUNpl_1_compare115/1 -> DSMR_ClntUsTElecMin/1
  DFC_BattUNpl_117/1 -> DFC_BattUNpl_1_compare116/1
  DFC_ClntUsTElecSig/1 -> DFC_BattUNpl_117/1
  DFC_BattUNpl_1_compare116/1 -> DSMR_ClntUsTElecSig/1
  DFC_BattUNpl_118/1 -> DFC_BattUNpl_1_compare117/1
  DFC_CoolPerfPlaus/1 -> DFC_BattUNpl_118/1
  DFC_BattUNpl_1_compare117/1 -> DSMR_CoolPerfPlaus/1
  DFC_BattUNpl_127/1 -> DFC_BattUNpl_1_compare126/1
  DFC_HtgPerfPlaus/1 -> DFC_BattUNpl_127/1
  DFC_BattUNpl_1_compare126/1 -> DSMR_HtgPerfPlaus/1
  DFC_BattUNpl_135/1 -> DFC_BattUNpl_1_compare127/1
  DFC_DChrgFobd/1 -> DFC_BattUNpl_135/1
  DFC_BattUNpl_1_compare127/1 -> DSMR_DChrgFobd/1
  DFC_BattUNpl_136/1 -> DFC_BattUNpl_1_compare134/1
  DFC_DChrgHvOnFail/1 -> DFC_BattUNpl_136/1
  DFC_BattUNpl_1_compare134/1 -> DSMR_DChrgHvOnFail/1
  DFC_BattUNpl_137/1 -> DFC_BattUNpl_1_compare135/1
  DFC_AChgHVOnTmt/1 -> DFC_BattUNpl_137/1
  DFC_BattUNpl_1_compare135/1 -> DSMR_AChgHVOnTmt/1
  DFC_BattUNpl_138/1 -> DFC_BattUNpl_1_compare136/1
  DFC_AChgHVOffTmt/1 -> DFC_BattUNpl_138/1
  DFC_BattUNpl_1_compare136/1 -> DSMR_AChgHVOffTmt/1
  DFC_BattUNpl_139/1 -> DFC_BattUNpl_1_compare137/1
  DFC_AChgS2ClsdTmt/1 -> DFC_BattUNpl_139/1
  DFC_BattUNpl_1_compare137/1 -> DSMR_AChgS2ClsdTmt/1
  DFC_BattUNpl_140/1 -> DFC_BattUNpl_1_compare138/1
  DFC_DChrgStakeErr/1 -> DFC_BattUNpl_140/1
  DFC_BattUNpl_1_compare138/1 -> DSMR_DChrgStakeErr/1
  DFC_BattUNpl_141/1 -> DFC_BattUNpl_1_compare139/1
  DFC_DChrgStkVoltErr/1 -> DFC_BattUNpl_141/1
  DFC_BattUNpl_1_compare139/1 -> DSMR_DChrgStkVoltErr/1
  DFC_BattUNpl_142/1 -> DFC_BattUNpl_1_compare140/1
  DFC_DChrgStkCurrErr/1 -> DFC_BattUNpl_142/1
  DFC_BattUNpl_1_compare140/1 -> DSMR_DChrgStkCurrErr/1
  DFC_BattUNpl_128/1 -> DFC_BattUNpl_1_compare141/1
  DFC_AChgPileRdyTmt/1 -> DFC_BattUNpl_128/1
  DFC_BattUNpl_1_compare141/1 -> DSMR_AChgPileRdyTmt/1
  DFC_BattUNpl_129/1 -> DFC_BattUNpl_1_compare128/1
  DFC_DChrgCHMTmt/1 -> DFC_BattUNpl_129/1
  DFC_BattUNpl_1_compare128/1 -> DSMR_DChrgCHMTmt/1
  DFC_BattUNpl_130/1 -> DFC_BattUNpl_1_compare129/1
  DFC_DChrgCRMTmt/1 -> DFC_BattUNpl_130/1
  DFC_BattUNpl_1_compare129/1 -> DSMR_DChrgCRMTmt/1
  DFC_BattUNpl_131/1 -> DFC_BattUNpl_1_compare130/1
  DFC_DChrgCMLTmt/1 -> DFC_BattUNpl_131/1
  DFC_BattUNpl_1_compare130/1 -> DSMR_DChrgCMLTmt/1
  DFC_BattUNpl_132/1 -> DFC_BattUNpl_1_compare131/1
  DFC_DChrgCROTmt/1 -> DFC_BattUNpl_132/1
  DFC_BattUNpl_1_compare131/1 -> DSMR_DChrgCROTmt/1
  DFC_BattUNpl_133/1 -> DFC_BattUNpl_1_compare132/1
  DFC_DChrgCCSTmt/1 -> DFC_BattUNpl_133/1
  DFC_BattUNpl_1_compare132/1 -> DSMR_DChrgCCSTmt/1
  DFC_BattUNpl_134/1 -> DFC_BattUNpl_1_compare133/1
  DFC_DChrgCSTTmt/1 -> DFC_BattUNpl_134/1
  DFC_BattUNpl_1_compare133/1 -> DSMR_DChrgCSTTmt/1
  DFC_BattUNpl_150/1 -> DFC_BattUNpl_1_compare148/1
  DFC_DChrgCSDTmt/1 -> DFC_BattUNpl_150/1
  DFC_BattUNpl_1_compare148/1 -> DSMR_DChrgCSDTmt/1
  DFC_BattUNpl_151/1 -> DFC_BattUNpl_1_compare149/1
  DFC_DChrgParaChk/1 -> DFC_BattUNpl_151/1
  DFC_BattUNpl_1_compare149/1 -> DSMR_DChrgParaChk/1
  DFC_BattUNpl_143/1 -> DFC_BattUNpl_1_compare150/1
  DFC_DChrgCableChk/1 -> DFC_BattUNpl_143/1
  DFC_BattUNpl_1_compare150/1 -> DSMR_DChrgCableChk/1
  DFC_BattUNpl_144/1 -> DFC_BattUNpl_1_compare142/1
  DFC_DChrgSLACTOut/1 -> DFC_BattUNpl_144/1
  DFC_BattUNpl_1_compare142/1 -> DSMR_DChrgSLACTOut/1
  DFC_BattUNpl_145/1 -> DFC_BattUNpl_1_compare143/1
  DFC_DChrgCnntErr/1 -> DFC_BattUNpl_145/1
  DFC_BattUNpl_1_compare143/1 -> DSMR_DChrgCnntErr/1
  DFC_BattUNpl_146/1 -> DFC_BattUNpl_1_compare144/1
  DFC_DChrgLckErr/1 -> DFC_BattUNpl_146/1
  DFC_BattUNpl_1_compare144/1 -> DSMR_DChrgLckErr/1
  DFC_BattUNpl_147/1 -> DFC_BattUNpl_1_compare145/1
  DFC_AChrgCnntErr/1 -> DFC_BattUNpl_147/1
  DFC_BattUNpl_1_compare145/1 -> DSMR_AChrgCnntErr/1
  DFC_BattUNpl_148/1 -> DFC_BattUNpl_1_compare146/1
  DFC_AChgLckTmt/1 -> DFC_BattUNpl_148/1
  DFC_BattUNpl_1_compare146/1 -> DSMR_AChgLckTmt/1
  DFC_BattUNpl_149/1 -> DFC_BattUNpl_1_compare147/1
  DFC_AChgRdyPndiTmt/1 -> DFC_BattUNpl_149/1
  DFC_BattUNpl_1_compare147/1 -> DSMR_AChgRdyPndiTmt/1
  DFC_BattUNpl_152/1 -> DFC_BattUNpl_1_compare151/1
  DFC_AChgRdyTmt/1 -> DFC_BattUNpl_152/1
  DFC_BattUNpl_1_compare151/1 -> DSMR_AChgRdyTmt/1
  DFC_BattUNpl_153/1 -> DFC_BattUNpl_1_compare152/1
  DFC_AChgingErr/1 -> DFC_BattUNpl_153/1
  DFC_BattUNpl_1_compare152/1 -> DSMR_AChgingErr/1
  DFC_BattUNpl_154/1 -> DFC_BattUNpl_1_compare153/1
  DFC_AChgUnlckTmt/1 -> DFC_BattUNpl_154/1
  DFC_BattUNpl_1_compare153/1 -> DSMR_AChgUnlckTmt/1
  DFC_BattUNpl_155/1 -> DFC_BattUNpl_1_compare154/1
  DFC_AChgFobd/1 -> DFC_BattUNpl_155/1
  DFC_BattUNpl_1_compare154/1 -> DSMR_AChgFobd/1
  DFC_BattUNpl_156/1 -> DFC_BattUNpl_1_compare155/1
  DFC_SocValJmp/1 -> DFC_BattUNpl_156/1
  DFC_BattUNpl_1_compare155/1 -> DSMR_SocValJmp/1
  DFC_BattUNpl_1_compare/1 -> DSMR_CurrRngErr/1
  DFC_BattUNpl_1/1 -> DFC_BattUNpl_1_compare/1
